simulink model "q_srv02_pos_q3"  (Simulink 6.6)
settings: Solver=ode1  StartTime=0.0  StopTime=inf  FixedStep=0.002  RelTol=1e-3  AbsTol=1e-6
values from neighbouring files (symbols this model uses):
  IMAX_AMP = 0    [config_srv02.m]
  K_ENC = 0    [config_srv02.m]
  K_POT = -(352 * pi / 180 / 10)    (= -0.614355896702)    [config_srv02.m]
  K_TACH = -(1000 * 2 * pi / 60 / 1.5 / Kg)    [config_srv02.m]
  ki = -( -AmpMax + kp * e_ss ) / ti / e_ss    [d_i_design.m]    (also in setup_srv02_exp02_pos.m = 0; d_pi_design.m = wn^2*tau/K; setup_srv02_exp03_spd.m = 0)
  kp = wn^2/K*tau    [d_pv_design.m]    (also in setup_srv02_exp02_pos.m = 0; d_pi_design.m = (-1+2*zeta*wn*tau)/K; setup_srv02_exp03_spd.m = 0)
  kv = (-1+2*zeta*wn*tau)/K    [d_pv_design.m]    (also in setup_srv02_exp02_pos.m = 0)
  VMAX_DAC = 10    [setup_srv02_exp02_pos.m]    (also in setup_srv02_exp01_mdl.m; setup_srv02_exp03_spd.m)
  wcf = 2 * pi * 50.0    (= 314.159265359)    [setup_srv02_exp02_pos.m]    (also in setup_srv02_exp03_spd.m)
  wcf_e = 2 * pi * 50.0    (= 314.159265359)    [setup_srv02_exp02_pos.m]    (also in setup_srv02_exp01_mdl.m = 157.079632679; setup_srv02_exp03_spd.m = 395.840674352)
  zetaf = 0.9    [setup_srv02_exp02_pos.m]    (also in setup_srv02_exp03_spd.m)
  zetaf_e = 0.9    [setup_srv02_exp02_pos.m]    (also in setup_srv02_exp01_mdl.m; setup_srv02_exp03_spd.m)
undefined symbols (not defined in the file or in its folder): HIL, qc_get_step_size, square
libraries: quarc_library x5

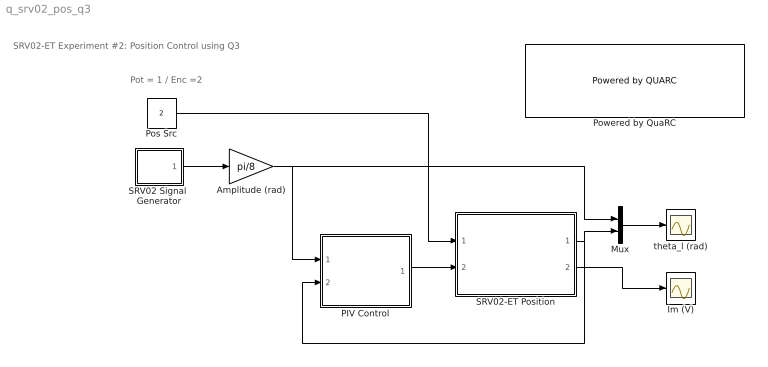
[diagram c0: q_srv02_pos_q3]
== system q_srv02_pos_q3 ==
  note: SRV02-ET Experiment #2: Position Control using Q3
  note: Pot = 1 / Enc =2
  Amplitude (rad) : Gain  Gain=pi/8
  Im (V) : Scope
  Mux : Mux  Inputs=2
  PIV Control : Subsystem
  Pos Src : Constant  Value=2
  Powered by QuaRC : quarc_library/Logos/Powered by QUARC  SystemSampleTime=-1
  SRV02 Signal  Generator : Subsystem  mask(QET Signal Generator){sig_type=square, a=1, f=0.4}
      mask prompts: sig_type "Signal Type"; a "Amplitude"; f "Frequency (Hz)"
      mask help: Generates a square, triangular, or sinusoidal waveform of a specified amplitude and frequency.
  SRV02-ET Position : Subsystem
  theta_l (rad) : Scope
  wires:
  Amplitude (rad)/1 -> Mux/1, PIV Control/1(theta_d (rad))
  SRV02-ET Position/1(theta_l (rad)) -> Mux/2, PIV Control/2(theta_l (rad))
  SRV02-ET Position/2(Im (V)) -> Im (V)/1
  Mux/1 -> theta_l (rad)/1
  PIV Control/1(u) -> SRV02-ET Position/2(I_ref (A))
  SRV02 Signal  Generator/1(out) -> Amplitude (rad)/1
  Pos Src/1 -> SRV02-ET Position/1(pos src)

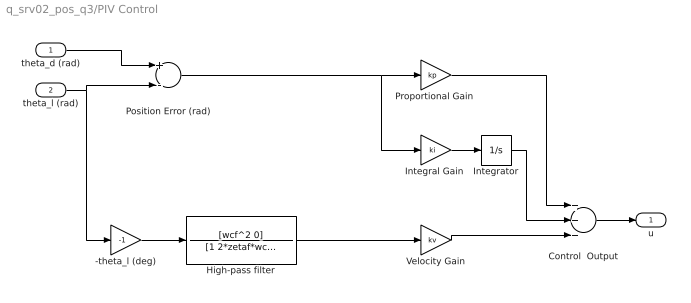
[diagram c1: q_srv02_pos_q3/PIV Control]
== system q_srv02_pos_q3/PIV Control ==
  theta_d (rad) : Inport
  theta_l (rad) : Inport  Port=2
  -theta_l (deg) : Gain  Gain=-1
  Control  Output : Sum  Inputs=+++  OutScaling=2^-10
  High-pass filter : TransferFcn  Numerator=[wcf^2 0]  Denominator=[1 2*zetaf*wcf wcf^2]
  "Integral Gain " : Gain  Gain=ki
  Integrator : Integrator  LimitOutput=on  UpperSaturationLimit=VMAX_DAC  LowerSaturationLimit=-VMAX_DAC
  Position Error (rad) : Sum  Inputs=+-  OutScaling=2^-10
  "Proportional Gain " : Gain  Gain=kp
  Velocity Gain : Gain  Gain=kv
  u : Outport
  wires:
  Integrator/1 -> Control  Output/2
  Velocity Gain/1 -> Control  Output/3
  "Integral Gain "/1 -> Integrator/1
  -theta_l (deg)/1 -> High-pass filter/1
  Position Error (rad)/1 -> "Proportional Gain "/1, "Integral Gain "/1
  theta_l (rad)/1 -> -theta_l (deg)/1, Position Error (rad)/2
  Control  Output/1 -> u/1
  theta_d (rad)/1 -> Position Error (rad)/1
  "Proportional Gain "/1 -> Control  Output/1
  High-pass filter/1 -> Velocity Gain/1

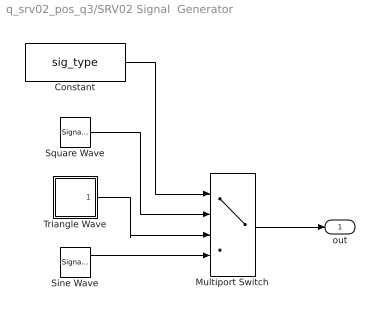
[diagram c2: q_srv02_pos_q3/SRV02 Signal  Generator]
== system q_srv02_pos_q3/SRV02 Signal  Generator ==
  Constant : Constant  Value=sig_type
  Multiport Switch : MultiPortSwitch  Inputs=3
  Sine Wave : SignalGenerator  Amplitude=a  Frequency=f
  Square Wave : SignalGenerator  WaveForm=square  Amplitude=a  Frequency=f
  Triangle Wave : Subsystem
  out : Outport
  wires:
  Constant/1 -> Multiport Switch/1
  Multiport Switch/1 -> out/1
  Sine Wave/1 -> Multiport Switch/4
  Triangle Wave/1(out) -> Multiport Switch/3
  Square Wave/1 -> Multiport Switch/2

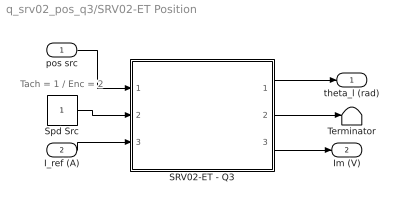
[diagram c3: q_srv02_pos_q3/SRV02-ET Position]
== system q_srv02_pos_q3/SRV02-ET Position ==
  note: Tach = 1 / Enc = 2
  pos src : Inport
  I_ref (A) : Inport  Port=2
  SRV02-ET - Q3 : Subsystem
  Spd Src : Constant
  Terminator : Terminator
  theta_l (rad) : Outport
  Im (V) : Outport  Port=2
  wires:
  SRV02-ET - Q3/2(omega_l (rad/s)) -> Terminator/1
  SRV02-ET - Q3/1(theta_l (rad)) -> theta_l (rad)/1
  I_ref (A)/1 -> SRV02-ET - Q3/3(I_ref (A))
  SRV02-ET - Q3/3(Im (A)) -> Im (V)/1
  Spd Src/1 -> SRV02-ET - Q3/2(spd src)
  pos src/1 -> SRV02-ET - Q3/1(pos src)

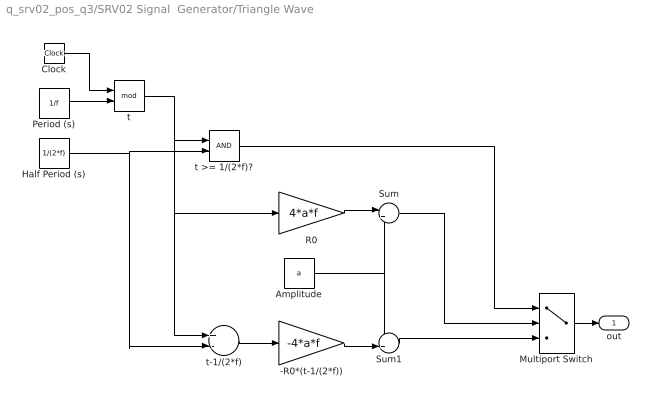
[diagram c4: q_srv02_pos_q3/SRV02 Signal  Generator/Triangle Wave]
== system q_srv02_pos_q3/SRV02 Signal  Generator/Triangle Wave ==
  -R0*(t-1/(2*f)) : Gain  Gain=-4*a*f
  Amplitude : Constant  Value=a
  Clock : Clock
  Half Period (s) : Constant  Value=1/(2*f)
  Multiport Switch : MultiPortSwitch  Inputs=2  zeroidx=on
  Period (s) : Constant  Value=1/f
  R0 : Gain  Gain=4*a*f
  Sum : Sum  Inputs=|+-
  Sum1 : Sum  Inputs=++|
  t : Math  Operator=mod
  t >= 1/(2*f)? : RelationalOperator  LogicOutDataTypeMode=Boolean
  t-1/(2*f) : Sum  Inputs=+-  OutScaling=2^-10
  out : Outport
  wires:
  Multiport Switch/1 -> out/1
  Clock/1 -> t/1
  Period (s)/1 -> t/2
  t/1 -> t >= 1/(2*f)?/1, R0/1, t-1/(2*f)/1
  Half Period (s)/1 -> t >= 1/(2*f)?/2, t-1/(2*f)/2
  t-1/(2*f)/1 -> -R0*(t-1/(2*f))/1
  R0/1 -> Sum/1
  Amplitude/1 -> Sum/2, Sum1/1
  -R0*(t-1/(2*f))/1 -> Sum1/2
  t >= 1/(2*f)?/1 -> Multiport Switch/1
  Sum/1 -> Multiport Switch/2
  Sum1/1 -> Multiport Switch/3

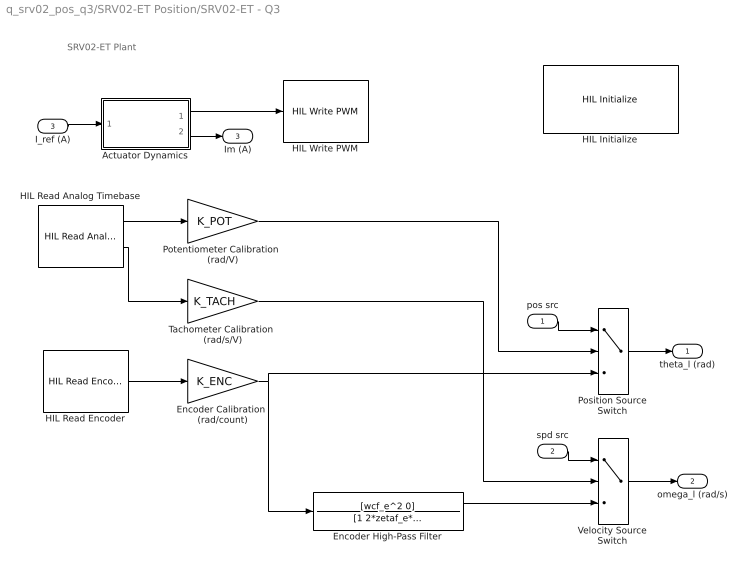
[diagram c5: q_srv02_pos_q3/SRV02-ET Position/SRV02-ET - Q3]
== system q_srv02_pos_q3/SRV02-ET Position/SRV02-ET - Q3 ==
  note: SRV02-ET Plant
  pos src : Inport
  spd src : Inport  Port=2
  I_ref (A) : Inport  Port=3
  Actuator Dynamics : Subsystem
  Encoder Calibration  (rad/count) : Gain  Gain=K_ENC
  Encoder High-Pass Filter : TransferFcn  Numerator=[wcf_e^2 0]  Denominator=[1 2*zetaf_e*wcf_e wcf_e^2]
  HIL Initialize : quarc_library/Data Acquisition/Generic/Configuration/HIL Initialize  object_name=HIL-1  board_type=q3_controlpaq_fw  board_number=0  exclusive=off  active=on  hardware_clocks=[]  clock_modes=[]  set_clock_params_at_start=off  set_clock_params_at_switch_in=off  analog_input_channels=0:1  analog_input_maximums=10  analog_input_minimums=-10  set_analog_input_params_at_start=off  set_analog_input_params_at_switch_in=off  analog_output_channels=[]  analog_output_maximums=[]  analog_output_minimums=[]  initial_analog_outputs=[]  final_analog_outputs=[]  watchdog_analog_outputs=0  set_analog_output_params_at_start=off  set_analog_output_params_at_switch_in=off  set_analog_outputs_at_start=off  set_analog_outputs_at_switch_in=off  set_analog_outputs_at_terminate=off  set_analog_outputs_at_switch_out=off  set_analog_outputs_on_watchdog=off  digital_input_channels=[]  digital_output_channels=[]  digital_output_configuration=[]  initial_digital_outputs=[]  final_digital_outputs=[]  watchdog_digital_outputs=0  set_digital_output_params_at_start=off  set_digital_output_params_at_switch_in=off  set_digital_outputs_at_start=off  set_digital_outputs_at_switch_in=off  set_digital_outputs_at_terminate=off  set_digital_outputs_at_switch_out=off  set_digital_outputs_on_watchdog=off  encoder_channels=0:2  quadrature=[]  encoder_filter_frequency=[]  initial_encoder_counts=0  set_encoder_params_at_start=off  set_encoder_params_at_switch_in=off  set_encoder_counts_at_start=on  set_encoder_counts_at_switch_in=off  pwm_channels=0:2  pwm_modes=[]  pwm_frequency=[]  pwm_configuration=[]  pwm_alignment=[]  pwm_polarity=[]  pwm_leading_deadband=[]  pwm_trailing_deadband=[]  initial_pwm_outputs=0  final_pwm_outputs=0  watchdog_pwm_outputs=0  set_pwm_params_at_start=off  set_pwm_params_at_switch_in=off  set_pwm_outputs_at_start=on  set_pwm_outputs_at_switch_in=off  set_pwm_outputs_at_terminate=on  set_pwm_outputs_at_switch_out=off  set_pwm_outputs_on_watchdog=off  other_output_channels=[]  initial_other_outputs=[]  final_other_outputs=[]  watchdog_other_outputs=0  set_other_outputs_at_start=off  set_other_outputs_at_switch_in=off  set_other_outputs_at_terminate=off  set_other_outputs_at_switch_out=off  set_other_outputs_on_watchdog=off
  HIL Read Analog Timebase : quarc_library/Data Acquisition/Generic/Timebases/HIL Read Analog Timebase  Tag=unassigned  object_name=HIL-1  clock=0  channels=[0:1]  samples_in_buffer=max(ceil(1/qc_get_step_size), 1)  active=on  vector_output=off
  HIL Read Encoder : quarc_library/Data Acquisition/Generic/Immediate I//O/HIL Read Encoder  Tag=unassigned  object_name=HIL-1  channels=0  sample_time=qc_get_step_size  active=on  vector_output=off  data_type_mode=Inherit via back propagation  data_type=double
  HIL Write PWM : quarc_library/Data Acquisition/Generic/Immediate I//O/HIL Write PWM  object_name=HIL-1  channels=0  sample_time=-1  active=off  vector_input=off
  Position Source Switch : MultiPortSwitch  Inputs=2
  Potentiometer Calibration  (rad/V) : Gain  Gain=K_POT
  Tachometer Calibration  (rad/s/V) : Gain  Gain=K_TACH
  Velocity Source Switch : MultiPortSwitch  Inputs=2
  theta_l (rad) : Outport  InitialOutput=0
  omega_l (rad/s) : Outport  Port=2  InitialOutput=0
  Im (A) : Outport  Port=3  InitialOutput=0
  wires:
  Position Source Switch/1 -> theta_l (rad)/1
  Potentiometer Calibration  (rad/V)/1 -> Position Source Switch/2
  pos src/1 -> Position Source Switch/1
  HIL Read Analog Timebase/1 -> Potentiometer Calibration  (rad/V)/1
  HIL Read Analog Timebase/2 -> Tachometer Calibration  (rad/s/V)/1
  Actuator Dynamics/1(Vdaq (V)) -> HIL Write PWM/1
  Tachometer Calibration  (rad/s/V)/1 -> Velocity Source Switch/2
  Encoder Calibration  (rad/count)/1 -> Position Source Switch/3, Encoder High-Pass Filter/1
  I_ref (A)/1 -> Actuator Dynamics/1(I_ref (A))
  Actuator Dynamics/2(Im (A)) -> Im (A)/1
  Velocity Source Switch/1 -> omega_l (rad/s)/1
  spd src/1 -> Velocity Source Switch/1
  Encoder High-Pass Filter/1 -> Velocity Source Switch/3
  HIL Read Encoder/1 -> Encoder Calibration  (rad/count)/1

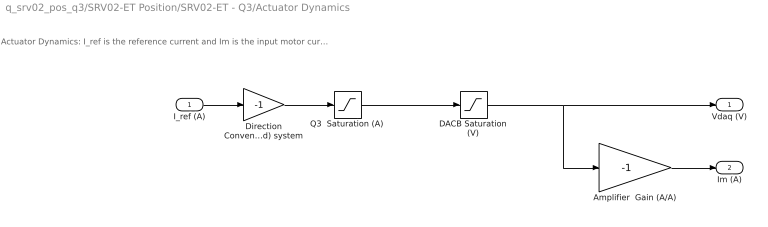
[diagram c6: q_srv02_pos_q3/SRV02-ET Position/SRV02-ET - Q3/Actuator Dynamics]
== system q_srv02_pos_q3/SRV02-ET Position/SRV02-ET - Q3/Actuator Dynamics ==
  note: Actuator Dynamics: I_ref is the reference current and Im is the input motor current after going through the DACB and Q3 amplifier limitations.
  I_ref (A) : Inport
  Amplifier  Gain (A/A) : Gain  Gain=-1
  DACB Saturation (V) : Saturate  UpperLimit=VMAX_DAC  LowerLimit=-VMAX_DAC
  Direction Convention: (Right-Hand) system : Gain  Gain=-1
  Q3  Saturation (A) : Saturate  UpperLimit=IMAX_AMP  LowerLimit=-IMAX_AMP
  Vdaq (V) : Outport
  Im (A) : Outport  Port=2
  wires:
  I_ref (A)/1 -> Direction Convention: (Right-Hand) system/1
  Q3  Saturation (A)/1 -> DACB Saturation (V)/1
  DACB Saturation (V)/1 -> Amplifier  Gain (A/A)/1, Vdaq (V)/1
  Amplifier  Gain (A/A)/1 -> Im (A)/1
  Direction Convention: (Right-Hand) system/1 -> Q3  Saturation (A)/1
